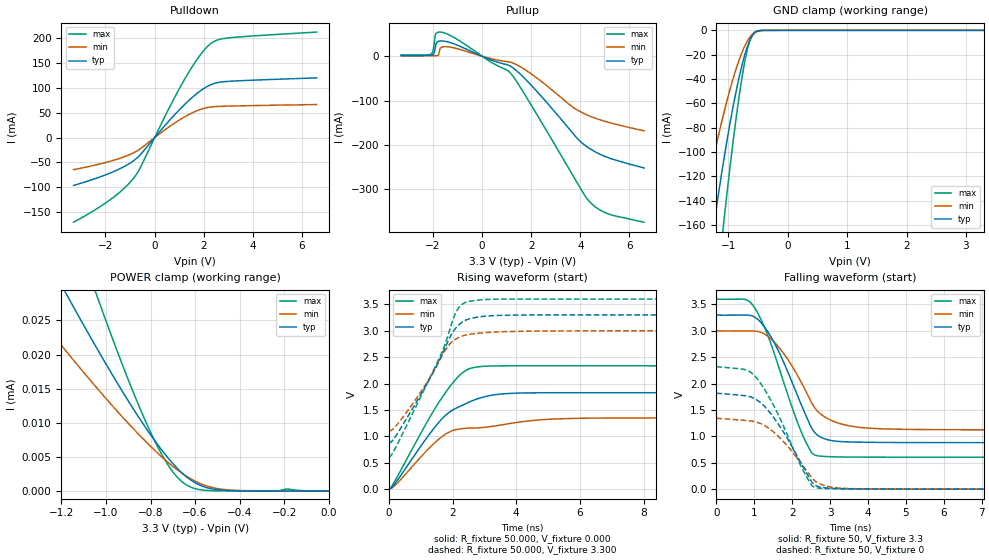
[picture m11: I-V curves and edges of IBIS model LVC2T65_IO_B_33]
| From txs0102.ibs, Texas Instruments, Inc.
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[Model]   LVC2T65_IO_B_33
Model_type  I/O
Vinl=0.15
Vinh=3.2
Enable   Active-High
Vref =   3.3
Rref =   1000000
Cref =   15p
Vmeas =   1.65
| variable   typ   min   max
C_comp   6.97pF   6.02pF   7.77pF
| C_pullup   6.85pF   5.99pF   7.78pF
| C_pulldown   7.55pF   6.65pF   8.48pF
| C_tri-state   6.97pF   6.02pF   7.77pF
[Temperature Range]   40   100   -40
| Ambient temperature   25   85   -40
[Voltage range]   3.3   3   3.6
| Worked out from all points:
|   slope of the pulldown table from 0 to 0.495 V, typ, clamps not added: 17.3 ohm
|   slope of the pullup table from 0 to 0.495 V, typ, clamps not added: 45.6 ohm
|   GND clamp passes 1 mA (typ) near -0.52 V on its own axis
|   rising waveform, R_fixture 50.000, V_fixture 0.000: 20-80 % time 1.4ns typ, 1.37ns min, 1.34ns max; typ from 0.004 V to 1.82 V
|   falling waveform, R_fixture 50, V_fixture 3.3: 20-80 % time 887ps typ, 935ps min, 866ps max; typ from 3.3 V to 0.88 V
|   rising waveform, R_fixture 50.000, V_fixture 3.300: 20-80 % time 1.29ns typ, 1.17ns min, 1.35ns max; typ from 0.87 V to 3.3 V
|   falling waveform, R_fixture 50, V_fixture 0: 20-80 % time 925ps typ, 939ps min, 914ps max; typ from 1.82 V to 0.004 V
[GND Clamp]
| LVC2T65_IO_B_33
|   Voltage   I(typ)   I(min)   I(max)
-3.3V     -1.072A    -772.9mA   -1.425A
-1.5V     -254.2mA   -167mA     -369.6mA
-1.45V    -235.1mA   -153.9mA   -343mA
-1.25V    -162.9mA   -105.2mA   -240.4mA
-1.225V   -154.4mA   -99.58mA   -228.1mA
-1.095V   -112.5mA   -71.94mA   -166.5mA
-1.075V   -106.4mA   -67.97mA   -157.4mA
-900mV    -57.96mA   -36.67mA   -84.13mA
-745mV    -24.17mA   -15.3mA    -31.73mA
-645mV    -9.129mA   -6.063mA   -9.578mA
-530mV    -1.302mA   -1.057mA   -747.9uA
3.3V      387.2pA    8.863nA    78.27pA
[POWER Clamp]
| LVC2T65_IO_B_33
|   Voltage   I(typ)   I(min)   I(max)
-3.3V     173.6uA    117.4uA    277.8uA
-1.395V   42.14uA    29.36uA    63.15uA
-1.35V    39.34uA    27.48uA    58.59uA
-1.2V     30.2uA     21.34uA    43.7uA
-1.15V    27.23uA    19.35uA    38.87uA
-1.05V    21.43uA    15.45uA    29.47uA
-795mV    8.01uA     6.39uA     8.27uA
-725mV    4.979uA    4.292uA    3.992uA
-660mV    2.678uA    2.627uA    1.384uA
-585mV    938.5nA    1.197uA    222.5nA
-495mV    158.4nA    316.7nA    13.56nA
0V        0A         0A         0A
[Pulldown]
| LVC2T65_IO_B_33
|   Voltage   I(typ)   I(min)   I(max)
-3.3V     -96.25mA   -64.56mA   -170.2mA
-1.745V   -70.06mA   -46.82mA   -122.8mA
-1.2V     -57.25mA   -38.02mA   -100.3mA
-830mV    -45.63mA   -30.04mA   -80.13mA
-585mV    -34.83mA   -22.75mA   -60.91mA
480mV     27.42mA    17.59mA    48.18mA
1.17V     63.85mA    40.08mA    112.6mA
1.81V     91.75mA    55.51mA    162.6mA
2.28V     106mA      61.29mA    188.6mA
2.575V    110.5mA    62.46mA    196.3mA
3.11V     113.3mA    63.35mA    200.8mA
6.6V      120mA      66.36mA    212mA
[Pullup]
| LVC2T65_IO_B_33
|   Voltage   I(typ)   I(min)   I(max)
-3.3V     1.65mA     889uA      2.704mA
-2.085V   2.407mA    904.5uA    4.707mA
-1.995V   3.798mA    960.4uA    13.69mA
-1.885V   25.66mA    1.169mA    50.48mA
-1.78V    33.47mA    3.189mA    54.2mA
-1.65V    34.53mA    20.22mA    54.13mA
1.06V     -19.92mA   -12.5mA    -32.8mA
1.735V    -50.01mA   -29.67mA   -85.74mA
3.625V    -168.9mA   -111.9mA   -261.7mA
4.345V    -206.7mA   -134mA     -325.9mA
5.16V     -229.1mA   -149.2mA   -355.8mA
6.6V      -251.9mA   -168.1mA   -374.1mA
[Ramp]
| LVC2T65_IO_B_33
| variable   typ   min   max
dV/dt_r   1.16/1.41E-09   0.87/1.39E-09   1.47/1.35E-09
dV/dt_f   1.45/8.87E-10   1.13/9.34E-10   1.80/8.66E-10
R_load = 50
[Rising Waveform]
R_fixture = 50.000
V_fixture = 0.000
V_fixture_min = 0.000
V_fixture_max = 0.000
C_fixture = 0.000
L_fixture = 0.000
|  time   V(typ)   V(min)   V(max)
0s        4.042mV    3.485mV    4.459mV
252ps     158.8mV    109.3mV    226.8mV
1.512ns   1.228V     920.5mV    1.593V
1.848ns   1.436V     1.07V      1.89V
2.1ns     1.533V     1.129V     2.082V
2.52ns    1.652V     1.16V      2.281V
3.528ns   1.803V     1.219V     2.337V
5.208ns   1.828V     1.331V     2.338V
8.652ns   1.828V     1.352V     2.337V
419.9ns   1.819V     1.345V     2.322V
[Falling Waveform]
| LVC2T65_IO_B_33
R_fixture =   50
C_fixture =   0
L_fixture =   0
V_fixture =   3.3
V_fixture_min = 3
V_fixture_max = 3.6
|   Time   V(typ)   V(min)   V(max)
0s        3.3V       3V         3.6V
756ps     3.297V     2.996V     3.594V
1.008ns   3.26V      2.994V     3.438V
1.344ns   2.996V     2.904V     2.937V
1.68ns    2.556V     2.66V      2.235V
2.184ns   1.698V     2.099V     1.184V
2.52ns    1.148V     1.626V     685.8mV
2.856ns   955.9mV    1.371V     622.2mV
3.444ns   898.6mV    1.211V     611.2mV
419.9ns   879.8mV    1.112V     607mV
[Rising Waveform]
R_fixture = 50.000
V_fixture = 3.300
V_fixture_min = 3.000
V_fixture_max = 3.600
C_fixture = 0.000
L_fixture = 0.000
|  time   V(typ)   V(min)   V(max)
0s        869.7mV    1.1V       600.7mV
168ps     965.6mV    1.164V     742.2mV
588ps     1.372V     1.486V     1.245V
1.512ns   2.35V      2.353V     2.392V
1.848ns   2.792V     2.703V     2.891V
2.016ns   2.982V     2.808V     3.222V
2.184ns   3.106V     2.87V      3.429V
2.52ns    3.226V     2.934V     3.557V
3.444ns   3.29V      2.979V     3.598V
419.9ns   3.3V       3V         3.6V
[Falling Waveform]
| LVC2T65_IO_B_33
R_fixture =   50
C_fixture =   0
L_fixture =   0
V_fixture =   0
V_fixture_min = 0
V_fixture_max = 0
|   Time   V(typ)   V(min)   V(max)
0s        1.819V     1.345V     2.322V
756ps     1.771V     1.305V     2.265V
1.092ns   1.681V     1.263V     2.078V
1.344ns   1.511V     1.175V     1.803V
1.68ns    1.186V     971.5mV    1.341V
2.184ns   562.4mV    542.9mV    508.3mV
2.52ns    135.8mV    214.6mV    70.05mV
2.856ns   30.19mV    71.12mV    15.77mV
3.444ns   10.31mV    17.22mV    6.869mV
419.9ns   3.924mV    3.314mV    4.373mV
